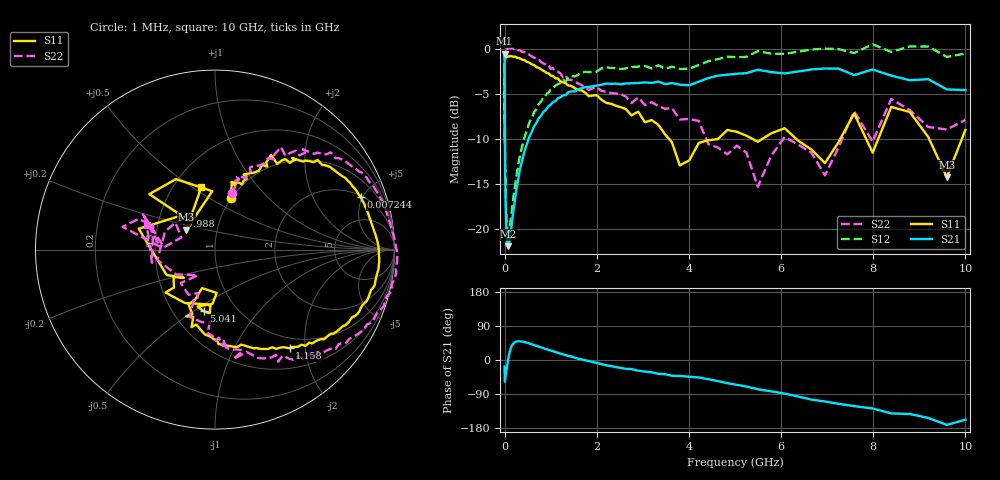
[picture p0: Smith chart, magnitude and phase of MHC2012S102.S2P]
!Agilent Technologies,E5071C,MY46111244,A.11.31
!Date: Tue May 07 16:55:33 2019
!Data & Calibration Information:
!Freq	S11:SOLT2(ON)	S21:SOLT2(ON)	S12:SOLT2(ON)	S22:SOLT2(ON)
# Hz S dB R 50
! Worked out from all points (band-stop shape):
!   201 points, 1 MHz to 10 GHz, reference 50 ohm
!   highest |S21| = -0.49 dB at 1.212 MHz (marker M1); lowest = -21.9 dB at 76.38 MHz (marker M2)
!   |S21| within 3 dB of the highest: start of sweep to 3.094 MHz; 4.266 GHz to 9.258 GHz (4.992 GHz wide, 73.8 % of centre)
!   lowest |S11| = -14.2 dB at 9.598 GHz (marker M3), VSWR 1.48, Z = 35.5 + j8.25 ohm
!   |S11| at or under -10 dB: start of sweep to 1.013 MHz; 3.578 GHz to 4.573 GHz (994.6 MHz wide, 24.4 % of centre); 6.341 GHz to 7.279 GHz (938.3 MHz wide, 13.8 % of centre)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
!   |S22| runs from -15.3 to 0.2 dB; largest |S21 - S12| = 0.45
!   S11 on the Smith chart (normalised r, x): 1 MHz: 1.00, +0.64; 7.244 MHz: 2.13, +4.86; 1.158 GHz: 0.82, -1.71; 5.041 GHz: 0.70, -0.55; 7.988 GHz: 0.64, +0.26; 10 GHz: 0.68, +0.55
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1000000  -10.34 72.6  -0.65 -17.3  0.81 -18.1  -9.69 72.7
1212171  -8.28 76.4  -0.49 -22.4  1.00 -23.4  -7.48 73.3
4810209  -1.72 29.7  -6.39 -54.6  -4.88 -55.4  -0.81 28.6
7244360  -1.28 19.7  -9.52 -57.2  -7.98 -58.0  -0.35 18.7
2.206931e7  -0.97 6.1  -16.82 -43.7  -15.28 -44.1  -0.05 5.4
7.638022e7  -0.79 -1.4  -21.88 0.7  -20.33 0.6  0.13 -1.3
1.047129e8  -0.76 -3.9  -21.49 17.6  -19.96 17.6  0.14 -4.6
4.810209e8  -1.38 -26.1  -10.63 45.8  -9.07 46.9  -0.50 -26.2
1.158214e9  -3.23 -52.8  -5.43 19.0  -3.84 23.0  -2.47 -54.6
2.206931e9  -5.94 -88.7  -3.79 -13.9  -1.97 -8.2  -4.72 -74.6
3.801894e9  -12.89 -108.6  -3.92 -42.1  -2.17 -32.5  -7.79 -94.2
5.041477e9  -9.16 -100.5  -2.70 -65.4  -0.86 -53.8  -10.70 -120.3
5.495409e9  -10.26 -95.8  -2.25 -77.2  -0.19 -64.0  -15.28 -123.6
6.078392e9  -8.76 -139.1  -2.66 -88.6  -0.49 -73.6  -9.73 -169.9
6.952868e9  -12.64 -137.8  -2.12 -109.5  0.10 -92.1  -14.01 160.2
7.585776e9  -7.12 164.7  -2.85 -121.7  -0.40 -105.8  -6.87 153.3
7.988146e9  -11.48 134.6  -2.23 -127.9  0.57 -111.1  -10.25 177.0
8.390517e9  -6.40 139.8  -2.91 -140.9  -0.28 -120.9  -5.51 166.1
8.792888e9  -6.95 119.0  -3.42 -142.5  0.34 -125.0  -6.73 158.3
9.195259e9  -9.75 92.7  -3.31 -152.9  0.32 -135.8  -8.63 158.3
9.597629e9  -14.22 144.9  -4.44 -171.2  -0.83 -151.5  -8.90 -168.2
1e10  -8.95 102.2  -4.52 -157.5  -0.46 -138.0  -7.84 159.9
